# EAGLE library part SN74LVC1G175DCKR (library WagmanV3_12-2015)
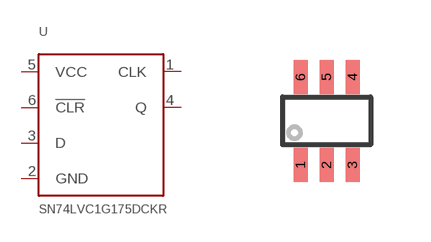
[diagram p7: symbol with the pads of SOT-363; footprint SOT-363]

Designator prefix U

## SN74LVC1G175DCKR  [SOT-363]
1  CLK
2  GND
3  D
4  Q
5  VCC
6  !CLR

## Footprint SOT-363 (pad centres in mm)
smd 0.35 x 0.85: 1 -0.65,-1.1; 2 0,-1.1; 3 0.65,-1.1; 4 0.65,1.1; 5 0,1.1; 6 -0.65,1.1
